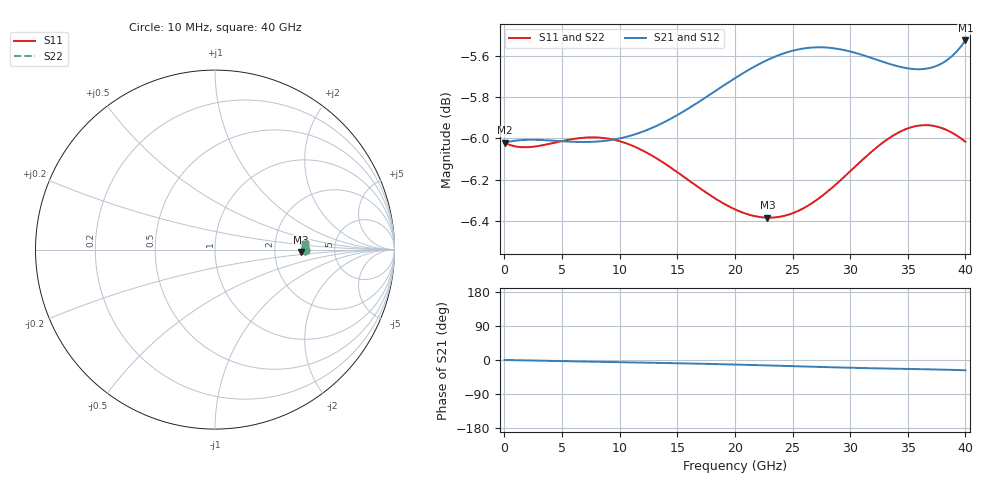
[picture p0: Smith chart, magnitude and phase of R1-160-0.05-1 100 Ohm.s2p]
!version-1
!date-09.2020
# MHz S RI R 50
!Freq ReS11 ImS11 ReS21 ImS21 ReS12 ImS12 ReS22 ImS22
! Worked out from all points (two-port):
!   101 points, 10 MHz to 40 GHz, reference 50 ohm
!   highest |S21| = -5.52 dB at 40 GHz (marker M1); lowest = -6.0 dB at 10 MHz (marker M2)
!   |S21| within 3 dB of the highest: start of sweep to end of sweep
!   lowest |S11| = -6.4 dB at 22.81 GHz (marker M3), VSWR 2.84, Z = 142 - j4.82 ohm
!   |S11| at or under -10 dB: nowhere
!   |S22| runs from -6.4 to -5.9 dB; largest |S21 - S12| = 0
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10  0.5 -6.71e-05  0.5 -4.05e-05  0.5 -4.05e-05  0.5 -6.71e-05
1210  0.4988 -0.00607  0.5006 -0.00546  0.5006 -0.00546  0.4988 -0.00607
2410  0.4988 -0.0089  0.5007 -0.0116  0.5007 -0.0116  0.4988 -0.0089
4010  0.4996 -0.00971  0.5002 -0.0203  0.5002 -0.0203  0.4996 -0.00971
6810  0.5013 -0.00812  0.4989 -0.0352  0.4989 -0.0352  0.5013 -0.00812
10010  0.5003 -0.00748  0.4986 -0.0508  0.4986 -0.0508  0.5003 -0.00748
11610  0.4983 -0.00841  0.4992 -0.0585  0.4992 -0.0585  0.4983 -0.00841
13610  0.4947 -0.0105  0.5007 -0.0684  0.5007 -0.0684  0.4947 -0.0105
16810  0.4875 -0.0144  0.5041 -0.0864  0.5041 -0.0864  0.4875 -0.0144
20010  0.4814 -0.0159  0.507 -0.108  0.507 -0.108  0.4814 -0.0159
21610  0.4797 -0.0148  0.5076 -0.1201  0.5076 -0.1201  0.4797 -0.0148
22810  0.4793 -0.0131  0.5074 -0.1295  0.5074 -0.1295  0.4793 -0.0131
24810  0.4803 -0.00837  0.5057 -0.1456  0.5057 -0.1456  0.4803 -0.00837
26810  0.4836 -0.00173  0.5021 -0.1612  0.5021 -0.1612  0.4836 -0.00173
28410  0.4875 0.00455  0.4981 -0.1729  0.4981 -0.1729  0.4875 0.00455
30010  0.492 0.0112  0.4932 -0.1833  0.4932 -0.1833  0.492 0.0112
31610  0.4965 0.0179  0.488 -0.1925  0.488 -0.1925  0.4965 0.0179
33610  0.5011 0.0253  0.4816 -0.2023  0.4816 -0.2023  0.5011 0.0253
35610  0.5036 0.031  0.4762 -0.2114  0.4762 -0.2114  0.5036 0.031
37610  0.5033 0.0341  0.4726 -0.2219  0.4726 -0.2219  0.5033 0.0341
38810  0.5017 0.0345  0.4715 -0.2304  0.4715 -0.2304  0.5017 0.0345
40000  0.4991 0.0337  0.4711 -0.2415  0.4711 -0.2415  0.4991 0.0337
